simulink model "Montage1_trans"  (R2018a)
settings: Solver=VariableStepAuto  StartTime=0.0  StopTime=2  RelTol=1e-3
model workspace: external: MATLAB File (data not in the file)
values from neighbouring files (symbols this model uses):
  smiData = struct    [Montage1_DataFile.m]    (also in Montage2_DataFile.m)
undefined symbols (not defined in the file or in its folder): kg, m, mm, N, s, X, Y, Z
libraries: sm_lib x10, nesl_utility x5

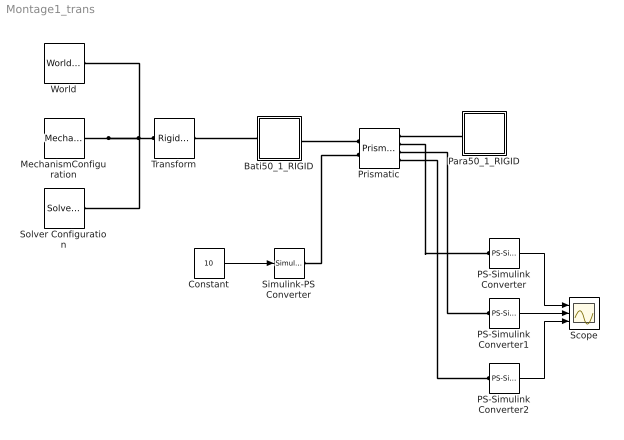
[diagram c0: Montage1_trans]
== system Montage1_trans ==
  Bati50_1_RIGID : Subsystem
  Constant : Constant  Value=10
  MechanismConfiguration : sm_lib/Utilities/Mechanism Configuration  UniformGravity=Constant  GravityVector=[0 -9.80665 0]  GravityUnits=m/s^2  LinearizationDelta=0.001
  PS-Simulink Converter : nesl_utility/PS-Simulink Converter  PhysicalDomain=network_engine_domain  SubClassName=ps_output  LeftPortType=input  RightPortType=output  PseudoPeriodic=off  Frequencies=[]  Unit=m  AffineConversion=off
  PS-Simulink Converter1 : nesl_utility/PS-Simulink Converter  PhysicalDomain=network_engine_domain  SubClassName=ps_output  LeftPortType=input  RightPortType=output  PseudoPeriodic=off  Frequencies=[]  Unit=m/s  AffineConversion=off
  PS-Simulink Converter2 : nesl_utility/PS-Simulink Converter  PhysicalDomain=network_engine_domain  SubClassName=ps_output  LeftPortType=input  RightPortType=output  PseudoPeriodic=off  Frequencies=[]  Unit=m/s^2  AffineConversion=off
  Para50_1_RIGID : Subsystem
  Prismatic : sm_lib/Joints/Prismatic Joint  SenseConstraintForce=off  SenseConstraintForceX=off  SenseConstraintForceY=off  SenseConstraintForceZ=off  SenseConstraintTorque=off  SenseConstraintTorqueX=off  SenseConstraintTorqueY=off  SenseConstraintTorqueZ=off  SenseTotalForce=off  SenseTotalForceX=off  SenseTotalForceY=off  SenseTotalForceZ=off  SenseTotalTorque=off  SenseTotalTorqueX=off  SenseTotalTorqueY=off  SenseTotalTorqueZ=off  CompositeWrenchDir=FollowerOnBase  CompositeWrenchFrame=BaseFrame  EquilibriumPosition=0  EquilibriumPositionUnits=m  SpringStiffness=0  SpringStiffnessUnits=N/m  DampingCoefficient=0  DampingCoefficientUnits=N/(m/s)  TorqueActuationMode=InputTorque  MotionActuationMode=ComputedMotion  SensePosition=on  SenseVelocity=on  SenseAcceleration=on  SenseTorqueForce=off  PositionTargetSpecify=on  PositionTargetPriority=Low  PositionTargetValue=smiData.PrismaticJoint(1).Pz.Pos  PositionTargetValueUnits=m  VelocityTargetSpecify=off  VelocityTargetPriority=High  VelocityTargetValue=0  VelocityTargetValueUnits=m/s
  Scope : Scope  NumInputPorts=3
  Simulink-PS Converter : nesl_utility/Simulink-PS Converter  PhysicalDomain=network_engine_domain  SubClassName=ps_input  LeftPortType=input  RightPortType=output  PseudoPeriodic=off  Frequencies=[]  NoiseDistribution=none  NoiseParameters=[]  Unit=A  AffineConversion=off  FilteringAndDerivatives=provide  SimscapeFilterOrder=1  InputFilterTimeConstant=0.001  UdotUserProvided=0
  Solver Configuration : nesl_utility/Solver Configuration  PhysicalDomain=network_engine_domain  SubClassName=solver  LeftPortType=input  RightPortType=generic  Tones=[]  Harmonics=[]  SimulateNoise=off  Profile=off  UseLocalSampling=off  EnableSwitchedLinearOptims=on  FrequencyDomain=off  UseCCode=off  RelTol=0.001  AbsTol=1e-06  MinStep=1e-09  ToWorkspace=off  RevertToSquareIcSolve=off  NumHomotopyIterations=100  PhasorMode=off  PhasorModeNumHarmonics=1  DoDC=off  ResidualTolerance=1e-09  UseLocalSolver=off  LocalSolverChoice=NE_BACKWARD_EULER_ADVANCER  LocalSolverSampleTime=0.001  DoFixedCost=off  MaxNonlinIter=3  MaxModeIter=2  LinearAlgebra=Sparse  EquationFormulation=NE_TIME_EF  DelaysMemoryBudget=1024  AutomaticFiltering=on  FilteringTimeConstant=0.001
  Transform : sm_lib/Frames and Transforms/Rigid Transform  TranslationMethod=Cartesian  TranslationStandardOffset=0  TranslationLengthUnit=mm  TranslationStandardAxis=+Z  TranslationCartesianOffset=smiData.RigidTransform(3).translation  TranslationROffset=0  TranslationROffsetUnits=m  TranslationZOffset=0  TranslationZOffsetUnits=m  TranslationThetaOffset=0  TranslationThetaOffsetUnits=deg  RotationMethod=ArbitraryAxis  RotationAngleUnits=rad  RotationStandardAxis=+Z  RotationAngle=smiData.RigidTransform(3).angle  RotationArbitraryAxis=smiData.RigidTransform(3).axis  FollAlignAxisA=+X  BaseAlignAxisA=+Y  FollAlignAxisB=+Y  BaseAlignAxisB=+Z  RotationSequenceAxes=FollowerAxes  RotationSequence=XYX  RotationSequenceAngles=[0 0 0]  RotationSequenceAnglesUnits=deg  RotationMatrix=[1 0 0; 0 1 0; 0 0 1]
  World : sm_lib/Frames and Transforms/World Frame
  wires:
  Constant/1 -> Simulink-PS Converter/1
  PS-Simulink Converter/1 -> Scope/1
  PS-Simulink Converter1/1 -> Scope/2
  PS-Simulink Converter2/1 -> Scope/3
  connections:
  Transform/LConn1 -- MechanismConfiguration/RConn1 -- Solver Configuration/RConn1 -- World/RConn1
  Bati50_1_RIGID/RConn1 -- Prismatic/LConn1
  Para50_1_RIGID/LConn1 -- Prismatic/RConn1
  Bati50_1_RIGID/LConn1 -- Transform/RConn1
  Simulink-PS Converter/RConn1 -- Prismatic/LConn2
  Prismatic/RConn2 -- PS-Simulink Converter/LConn1
  PS-Simulink Converter1/LConn1 -- Prismatic/RConn3
  PS-Simulink Converter2/LConn1 -- Prismatic/RConn4

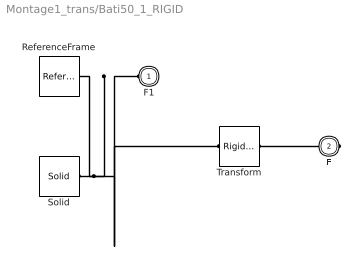
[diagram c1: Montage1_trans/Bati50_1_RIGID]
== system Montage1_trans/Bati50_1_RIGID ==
  ReferenceFrame : sm_lib/Frames and Transforms/Reference Frame
  Solid : sm_lib/Body Elements/Solid  InertiaType=Custom  Mass=smiData.Solid(2).mass  MassUnits=kg  CenterOfMass=smiData.Solid(2).CoM  CenterOfMassUnits=mm  MomentsOfInertia=smiData.Solid(2).MoI  MomentsOfInertiaUnits=kg*mm^2  ProductsOfInertia=smiData.Solid(2).PoI  ProductsOfInertiaUnits=kg*mm^2  DensityBased=on  Density=1000  DensityUnits=kg/m^3  DoExposeReferenceFrame=on  SerializedFrames=<Frames/>  GraphicType=FromGeometry  MarkerShape=Sphere  MarkerSize=10  GraphicVisPropType=SimpleVisualProperties  GraphicDiffuseColor=smiData.Solid(2).color  GraphicSpecularColor=[0.5 0.5 0.5 1.0]  GraphicAmbientColor=[0.15 0.15 0.15 1.0]  GraphicEmissiveColor=[0.0 0.0 0.0 1.0]  GraphicShininess=75  GraphicOpacity=smiData.Solid(2).opacity  GeometryShape=FromFile  RectangleSize=[1 1]  RectangleSizeUnits=m  BrickDimensions=[1 1 1]  BrickDimensionUnits=m  CylinderRadius=1  CylinderRadiusUnits=m  CylinderLength=1  CylinderLengthUnits=m  SphereRadius=1  SphereRadiusUnits=m  EllipsoidRadii=[1 1 1]  EllipsoidRadiiUnits=m  ExtrusionCrossSection=[1 1; -1 1; -1 -1; 1 -1]  ExtrusionCrossSectionUnits=m  ExtrusionLength=1  ExtrusionLengthUnits=m  PolygonNumSides=3  PolygonOuterRadius=1  PolygonOuterRadiusUnits=m  ExtGeomFileType=STEP  ExtGeomFileName=Bati50_Défaut_sldprt.STEP  ExtGeomFileUnits=m  RevolutionCrossSection=[1 1; 1 -1; 2 -1; 2 1]  RevolutionCrossSectionUnits=m  RevolutionExtent=Full  RevolutionAngle=180  RevolutionAngleUnits=deg
  Transform : sm_lib/Frames and Transforms/Rigid Transform  TranslationMethod=Cartesian  TranslationStandardOffset=0  TranslationLengthUnit=mm  TranslationStandardAxis=+Z  TranslationCartesianOffset=smiData.RigidTransform(1).translation  TranslationROffset=0  TranslationROffsetUnits=m  TranslationZOffset=0  TranslationZOffsetUnits=m  TranslationThetaOffset=0  TranslationThetaOffsetUnits=deg  RotationMethod=ArbitraryAxis  RotationAngleUnits=rad  RotationStandardAxis=+Z  RotationAngle=smiData.RigidTransform(1).angle  RotationArbitraryAxis=smiData.RigidTransform(1).axis  FollAlignAxisA=+X  BaseAlignAxisA=+Y  FollAlignAxisB=+Y  BaseAlignAxisB=+Z  RotationSequenceAxes=FollowerAxes  RotationSequence=XYX  RotationSequenceAngles=[0 0 0]  RotationSequenceAnglesUnits=deg  RotationMatrix=[1 0 0; 0 1 0; 0 0 1]
  F1 : PMIOPort  Side=Left
  F : PMIOPort  Port=2  Side=Right
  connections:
  Solid/RConn1 -- ReferenceFrame/RConn1 -- Transform/LConn1 -- F1/RConn1
  Transform/RConn1 -- F/RConn1

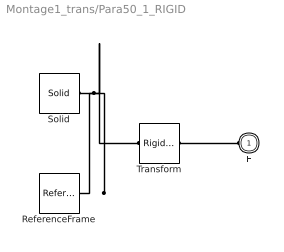
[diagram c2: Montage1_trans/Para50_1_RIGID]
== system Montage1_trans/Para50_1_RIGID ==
  ReferenceFrame : sm_lib/Frames and Transforms/Reference Frame
  Solid : sm_lib/Body Elements/Solid  InertiaType=Custom  Mass=smiData.Solid(1).mass  MassUnits=kg  CenterOfMass=smiData.Solid(1).CoM  CenterOfMassUnits=mm  MomentsOfInertia=smiData.Solid(1).MoI  MomentsOfInertiaUnits=kg*mm^2  ProductsOfInertia=smiData.Solid(1).PoI  ProductsOfInertiaUnits=kg*mm^2  DensityBased=on  Density=1000  DensityUnits=kg/m^3  DoExposeReferenceFrame=on  SerializedFrames=<Frames/>  GraphicType=FromGeometry  MarkerShape=Sphere  MarkerSize=10  GraphicVisPropType=SimpleVisualProperties  GraphicDiffuseColor=[1.0 0.0 0.2]  GraphicSpecularColor=[0.5 0.5 0.5 1.0]  GraphicAmbientColor=[0.15 0.15 0.15 1.0]  GraphicEmissiveColor=[0.0 0.0 0.0 1.0]  GraphicShininess=75  GraphicOpacity=smiData.Solid(1).opacity  GeometryShape=FromFile  RectangleSize=[1 1]  RectangleSizeUnits=m  BrickDimensions=[1 1 1]  BrickDimensionUnits=m  CylinderRadius=1  CylinderRadiusUnits=m  CylinderLength=1  CylinderLengthUnits=m  SphereRadius=1  SphereRadiusUnits=m  EllipsoidRadii=[1 1 1]  EllipsoidRadiiUnits=m  ExtrusionCrossSection=[1 1; -1 1; -1 -1; 1 -1]  ExtrusionCrossSectionUnits=m  ExtrusionLength=1  ExtrusionLengthUnits=m  PolygonNumSides=3  PolygonOuterRadius=1  PolygonOuterRadiusUnits=m  ExtGeomFileType=STEP  ExtGeomFileName=Para50_Défaut_sldprt.STEP  ExtGeomFileUnits=m  RevolutionCrossSection=[1 1; 1 -1; 2 -1; 2 1]  RevolutionCrossSectionUnits=m  RevolutionExtent=Full  RevolutionAngle=180  RevolutionAngleUnits=deg
  Transform : sm_lib/Frames and Transforms/Rigid Transform  TranslationMethod=Cartesian  TranslationStandardOffset=0  TranslationLengthUnit=mm  TranslationStandardAxis=+Z  TranslationCartesianOffset=smiData.RigidTransform(2).translation  TranslationROffset=0  TranslationROffsetUnits=m  TranslationZOffset=0  TranslationZOffsetUnits=m  TranslationThetaOffset=0  TranslationThetaOffsetUnits=deg  RotationMethod=ArbitraryAxis  RotationAngleUnits=rad  RotationStandardAxis=+Z  RotationAngle=smiData.RigidTransform(2).angle  RotationArbitraryAxis=smiData.RigidTransform(2).axis  FollAlignAxisA=+X  BaseAlignAxisA=+Y  FollAlignAxisB=+Y  BaseAlignAxisB=+Z  RotationSequenceAxes=FollowerAxes  RotationSequence=XYX  RotationSequenceAngles=[0 0 0]  RotationSequenceAnglesUnits=deg  RotationMatrix=[1 0 0; 0 1 0; 0 0 1]
  F : PMIOPort  Side=Left
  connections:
  Solid/RConn1 -- ReferenceFrame/RConn1 -- Transform/LConn1
  Transform/RConn1 -- F/RConn1
